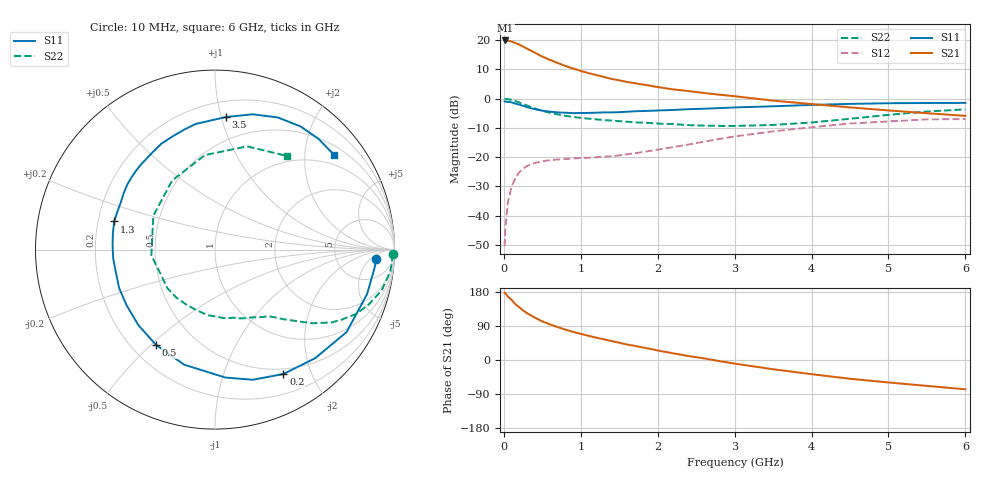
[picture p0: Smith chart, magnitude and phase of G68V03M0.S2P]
! SIEMENS Small Signal Semiconductors
! BFG193
! Si NPN RF Bipolar Junction Transistor in SOT223
! VCE = 8 V  IC = 3 mA
! Common Emitter S-Parameters:  August  1996
# GHz  S  MA  R  50
!  f  S11  S21  S12  S22
! GHz  MAG  ANG  MAG  ANG  MAG  ANG  MAG  ANG
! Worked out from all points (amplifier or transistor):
!   36 points, 10 MHz to 6 GHz, reference 50 ohm
!   highest |S21| = 19.9 dB at 20 MHz (marker M1)
!   |S21| within 3 dB of that: start of sweep to 316.3 MHz
!   unconditionally stable (mu >= 1): 1.299 GHz to 2.546 GHz
!   at 250 MHz: K = 0.23, MSG = 20.9 dB, |S12| = -23.9 dB
!   at 1.4 GHz: K = 1.07, MAG = 11.6 dB, |S12| = -19.7 dB
!   at 6 GHz: K = 0.90, MSG = 0.5 dB, |S12| = -7.0 dB
!   S11 on the Smith chart (normalised r, x): 10 MHz: 14, -8; 200 MHz: 0.43, -1.61; 500 MHz: 0.30, -0.52; 1.3 GHz: 0.27, +0.13; 3.5 GHz: 0.32, +1.04; 6 GHz: 0.72, +2.69
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0.01  0.8992 -3.4  9.907 177.4  0.003 93.2  0.9938 -1.5
0.02  0.8947 -6.6  9.915 176.2  0.0063 88.1  0.9893 -2.8
0.05  0.8829 -16.3  9.875 168.0  0.0161 79.5  0.9843 -7.1
0.1  0.8651 -32.1  9.496 158.7  0.0312 73.4  0.9562 -13.7
0.15  0.8233 -47.3  8.945 147.4  0.0441 64.5  0.9101 -19.6
0.2  0.791 -61.2  8.419 139.2  0.055 58.7  0.8643 -24.5
0.25  0.7552 -73.8  7.808 130.8  0.0637 52.6  0.8093 -28.7
0.3  0.715 -85.4  7.2 123.7  0.0705 48.5  0.7662 -32.0
0.4  0.6638 -105.0  6.161 112.3  0.0792 40.8  0.6815 -37.0
0.5  0.6244 -121.8  5.253 102.0  0.085 35.5  0.6189 -40.4
0.6  0.5995 -135.4  4.607 94.0  0.089 32.3  0.5742 -43.2
0.7  0.582 -147.7  4.085 86.7  0.0912 30.6  0.5397 -45.8
0.8  0.5756 -158.1  3.635 80.2  0.0931 28.9  0.5091 -48.1
1.1  0.5712 177.5  2.741 63.9  0.0979 28.8  0.4558 -55.6
1.3  0.5828 164.4  2.357 54.6  0.102 30.0  0.4312 -61.0
1.6  0.5983 148.2  1.934 40.9  0.1118 32.6  0.4045 -71.3
2.2  0.6414 123.8  1.444 17.7  0.1487 34.8  0.3678 -96.3
3  0.7083 98.7  1.102 -9.6  0.2261 27.0  0.3416 -140.7
3.5  0.7414 85.2  0.927 -24.4  0.2765 15.7  0.3559 -174.9
4.5  0.8151 64.6  0.71 -49.5  0.3759 -6.7  0.4533 121.7
5.5  0.8446 46.9  0.564 -68.3  0.4425 -34.7  0.6024 72.7
6  0.8475 38.6  0.509 -77.3  0.4486 -50.1  0.6578 52.5
